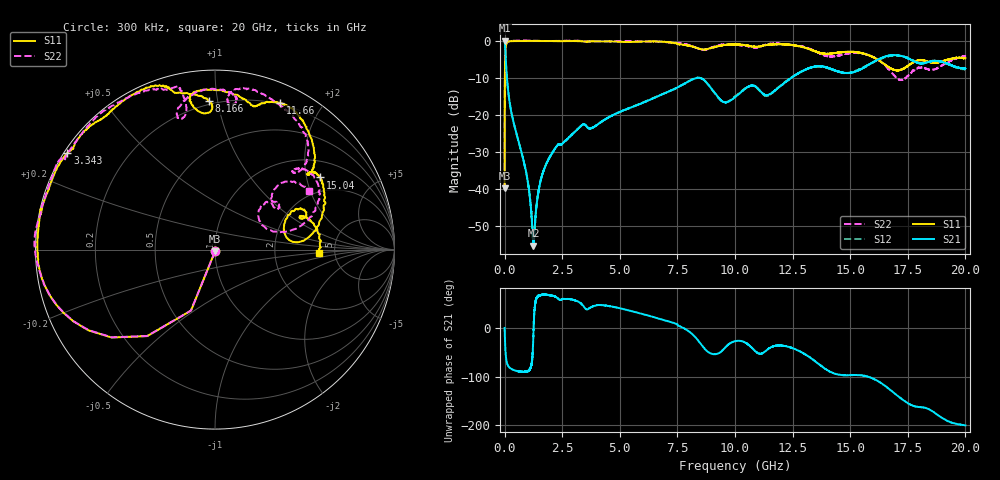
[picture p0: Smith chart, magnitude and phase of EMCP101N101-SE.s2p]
!EMCP101N101
!Johanson Technology Inc.
!www.johansontechnology.com
!Test Board Conditions:
!Substrate Type  RO4350B
!Substrate Thickness  10 mil
!Substrate Dk  3.66
!TL Type: GCPW
!TL Trace Width  20 mil
!TL Gap  10 mil
!PART MODE SINGLE ENDED (AKA BYPASS)
!DUT TOPOLOGY	SERIES-SHUNT
# MHz S  dB  R 50
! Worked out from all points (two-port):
!   20001 points, 300 kHz to 20 GHz, reference 50 ohm
!   highest |S21| = -0.01 dB at 300 kHz (marker M1); lowest = -55.3 dB at 1.252 GHz (marker M2)
!   |S21| within 3 dB of the highest: start of sweep to 33.53 MHz
!   lowest |S11| = -39.9 dB at 300 kHz (marker M3), VSWR 1.02, Z = 50 - j1.01 ohm
!   |S11| at or under -10 dB: start of sweep to 11.3 MHz
!   |S22| runs from -40.4 to 0.1 dB; largest |S21 - S12| = 0.017
!   S11 on the Smith chart (normalised r, x): 300 kHz: 1.00, -0.02; 3.343 GHz: 0.01, +0.30; 8.166 GHz: 0.18, +0.94; 11.66 GHz: 0.19, +1.52; 15.04 GHz: 1.49, +2.42; 20 GHz: 3.76, -0.19
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0.3  -39.88 -90.9  -0.01 -0.3  -0.01 -0.5  -40.39 -87.4
101.298  -0.49 -162.5  -10.11 -71.9  -10.06 -71.9  -0.52 -162.2
130.298  -0.32 -166.7  -12.16 -75.9  -12.12 -75.9  -0.35 -166.2
325.295  -0.11 -177.2  -20.24 -85.2  -20.21 -85.5  -0.06 -175.7
964.286  -0.06 172.6  -36.45 -89.1  -36.54 -89.4  0.06 175.1
1252.281  -0.06 169.3  -55.32 -12.2  -54.87 -13.6  0.01 171.7
1525.277  -0.08 168.4  -38.83 66.8  -38.84 67.1  -0.06 166.0
1835.272  -0.07 165.8  -32.93 67.4  -32.86 67.7  -0.09 161.5
3334.25  -0.15 146.9  -22.89 49.1  -22.91 49.2  -0.08 149.2
3343.25  -0.15 146.7  -22.86 48.7  -22.86 48.7  -0.08 149.2
6667.2  -0.20 111.6  -14.96 19.2  -14.92 18.8  -0.27 115.4
8166.178  -1.62 92.4  -10.42 -14.0  -10.39 -14.1  -1.53 101.3
8986.165  -1.93 98.5  -13.01 -53.2  -13.07 -53.0  -1.84 104.8
10000.15  -0.99 92.4  -15.27 -27.4  -15.08 -27.3  -1.06 85.3
10707.14  -1.50 77.0  -12.11 -39.9  -12.13 -41.0  -1.67 81.8
11656.12  -0.97 66.0  -13.83 -37.9  -13.84 -36.7  -0.77 78.6
13334.1  -2.55 42.1  -7.18 -63.6  -7.16 -63.9  -2.39 46.7
15043.07  -2.96 34.4  -8.63 -97.0  -8.51 -96.1  -3.31 38.8
16667.05  -7.11 5.4  -4.04 -124.7  -4.16 -124.4  -7.66 14.2
17214.04  -7.78 19.3  -4.09 -145.2  -4.11 -143.9  -10.56 31.2
17864.03  -5.49 25.2  -5.83 -161.7  -5.66 -161.4  -7.60 40.1
20000  -4.72 -1.7  -7.51 159.7  -7.70 160.8  -4.11 31.7
